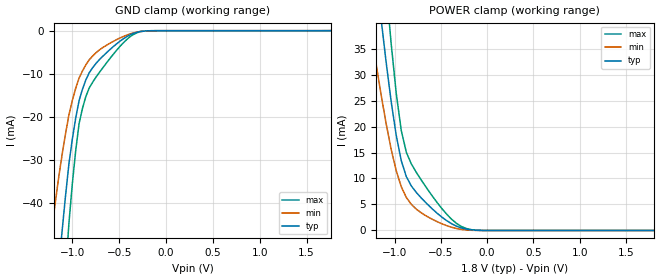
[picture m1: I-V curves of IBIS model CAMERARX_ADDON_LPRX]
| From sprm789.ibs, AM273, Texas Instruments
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|   Model Cell CAMERARX_ADDON_LPRX
|CAMERARX_ADDON_LPRX
[Model]   CAMERARX_ADDON_LPRX
Model_type   Input
Polarity   Non-Inverting
Vinl =  0.654
Vinh =  0.749
C_comp   4.13955p   3.54298p   4.784869p
[Model Spec]
Vinl   0.654   0.586   0.722
Vinh   0.749   0.675   0.822
[Temperature Range]   25   125   -40
[Voltage Range]   1.8   1.62   1.92
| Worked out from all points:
|   GND clamp passes 1 mA (typ) near -0.39 V on its own axis
|   POWER clamp passes 1 mA (typ) near -0.35 V on its own axis
[POWER_clamp]
|   voltage   I(typ)   I(min)   I(max)
-1.8V     156.8mA    109.4mA    217.7mA
-1.255V   58.58mA    38.5mA     83.58mA
-1.127V   37.93mA    24.29mA    54.73mA
-1.055V   27.33mA    17.27mA    39.59mA
-981.8mV  18.3mA     11.5mA     26.4mA
-927.3mV  13.42mA    8.419mA    19.22mA
-872.7mV  10.36mA    6.348mA    15.04mA
-818.2mV  8.551mA    5.012mA    12.79mA
-654.5mV  5.218mA    2.76mA     8.209mA
-381.8mV  1.281mA    612uA      2.13mA
-163.6mV  106uA      34.63uA    142.1uA
1.8V      2.655uA    1.447uA    5.48uA
[GND_clamp]
|   voltage   I(typ)   I(min)   I(max)
-1.8V     -252.1mA   -161mA     -379.9mA
-1.218V   -74.99mA   -46.16mA   -113.7mA
-1.109V   -46.67mA   -28.87mA   -69.57mA
-1.036V   -31.06mA   -19.64mA   -44.89mA
-963.6mV  -20.33mA   -13.39mA   -27.93mA
-927.3mV  -16.23mA   -11mA      -21.58mA
-854.5mV  -11.42mA   -7.916mA   -15.25mA
-818.2mV  -9.733mA   -6.736mA   -13.26mA
-636.4mV  -5.156mA   -3.402mA   -7.535mA
-418.2mV  -1.379mA   -1.021mA   -2.048mA
-272.7mV  -182.6uA   -178.1uA   -212.2uA
1.764V    1.345uA    26.47uA    2.07uA
